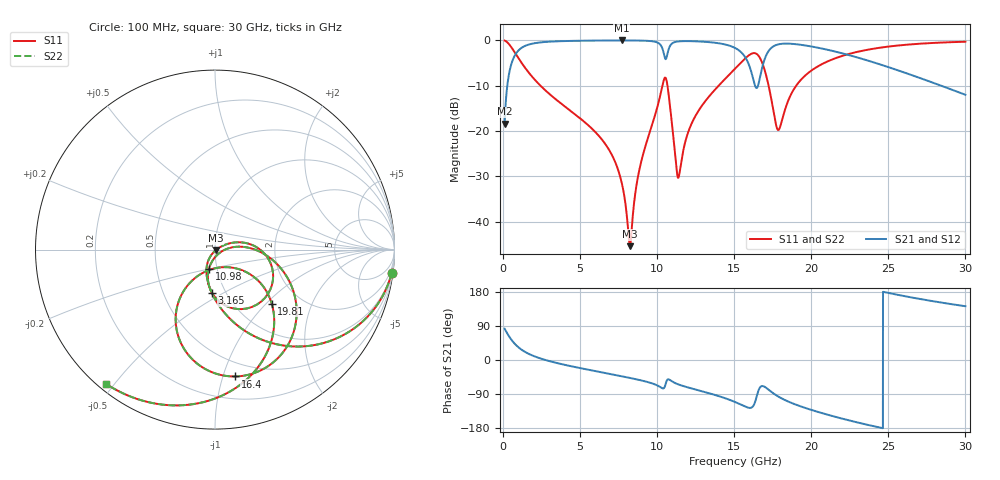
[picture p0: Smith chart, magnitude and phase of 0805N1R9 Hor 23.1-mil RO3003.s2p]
# GHz S MA R 50
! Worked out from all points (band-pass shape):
!   3201 points, 100 MHz to 30 GHz, reference 50 ohm
!   highest |S21| = -0.05 dB at 7.706 GHz (marker M1); lowest = -18.4 dB at 100 MHz (marker M2)
!   |S21| within 3 dB of the highest: 816.5 MHz to 10.44 GHz (9.624 GHz wide, 171 % of centre); 17.11 GHz to 22.19 GHz (5.078 GHz wide, 25.8 % of centre)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
!   lowest |S11| = -45.4 dB at 8.229 GHz (marker M3), VSWR 1.01, Z = 50.3 - j0.415 ohm
!   |S11| at or under -10 dB: 2.422 GHz to 10.34 GHz (7.919 GHz wide, 124 % of centre); 10.67 GHz to 13.99 GHz (3.326 GHz wide, 27 % of centre); 17.23 GHz to 19.03 GHz (1.797 GHz wide, 9.91 % of centre)
!   |S22| runs from -45.4 to -0.1 dB; largest |S21 - S12| = 0
!   S11 on the Smith chart (normalised r, x): 100 MHz: 1, -15; 3.165 GHz: 0.86, -0.44; 10.98 GHz: 0.91, -0.20; 16.4 GHz: 0.38, -1.10; 19.81 GHz: 1.45, -1.08; 30 GHz: 0.02, -0.48
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0.1  0.9927 -7.5  0.1206 82.5  0.1206 82.5  0.9927 -7.5
0.4176875  0.8916 -29.4  0.4525 60.6  0.4525 60.6  0.8916 -29.4
0.8475  0.6958 -50.9  0.7174 39.1  0.7174 39.1  0.6958 -50.9
3.16475  0.2426 -94.1  0.9679 -4.6  0.9679 -4.6  0.2426 -94.1
5.089563  0.1338 -110.9  0.9879 -22.1  0.9879 -22.1  0.1338 -110.9
7.705813  0.02651 -123.0  0.9948 -42.9  0.9948 -42.9  0.02651 -123.0
8.229062  0.005363 -50.2  0.9944 -47.3  0.9944 -47.3  0.005363 -50.2
8.855094  0.0381 26.3  0.9918 -52.8  0.9918 -52.8  0.0381 26.3
10.06978  0.2 8.4  0.9348 -68.3  0.9348 -68.3  0.2 8.4
10.54631  0.3852 -52.9  0.6188 -63.8  0.6188 -63.8  0.3852 -52.9
10.97612  0.113 -107.5  0.9242 -56.8  0.9242 -56.8  0.113 -107.5
11.39659  0.03107 -38.9  0.9716 -64.7  0.9716 -64.7  0.03107 -38.9
12.45244  0.1432 6.5  0.9744 -77.5  0.9744 -77.5  0.1432 6.5
15.05  0.4853 -26.9  0.8233 -110.8  0.8233 -110.8  0.4853 -26.9
15.83488  0.6582 -50.5  0.5964 -125.0  0.5964 -125.0  0.6582 -50.5
16.3955  0.7156 -81.0  0.303 -105.4  0.303 -105.4  0.7156 -81.0
16.98416  0.4627 -118.2  0.6257 -71.0  0.6257 -71.0  0.4627 -118.2
17.85312  0.1024 -81.4  0.9001 -96.3  0.9001 -96.3  0.1024 -81.4
19.80597  0.4365 -43.6  0.8656 -129.1  0.8656 -129.1  0.4365 -43.6
20.03956  0.4676 -46.0  0.8519 -132.1  0.8519 -132.1  0.4676 -46.0
25.01978  0.8522 -94.4  0.5044 176.8  0.5044 176.8  0.8522 -94.4
30  0.9634 -129.0  0.2506 141.9  0.2506 141.9  0.9634 -129.0
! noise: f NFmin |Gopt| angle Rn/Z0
0.1  0.001059  0.9441  1.423  0.004239
3.417  0.006657  0.718  20.88  0.004519
6.743  0.01191  0.6998  39.37  0.006912
10.06  0.04998  0.8858  56.98  0.07346
13.39  0.03476  0.7996  73.55  0.02323
16.7  0.3227  0.9715  89.6  1.298
20.03  0.05969  0.8342  103.7  0.02937
23.35  0.05916  0.8145  116.5  0.01895
26.67  0.07135  0.8308  128.8  0.01724
30  0.09331  0.8606  140.8  0.01686
